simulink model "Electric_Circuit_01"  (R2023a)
settings: Solver=VariableStepAuto  StartTime=0.0  StopTime=10.0  RelTol=1e-3
libraries: fl_lib x8

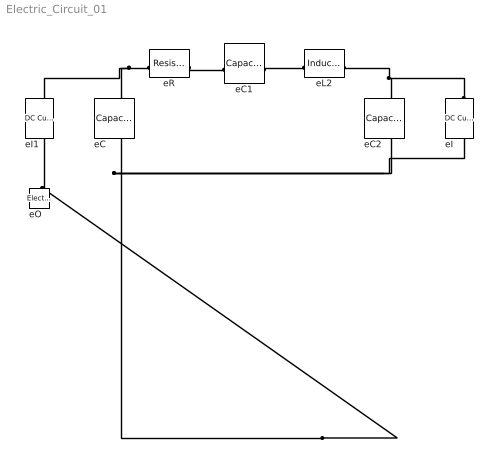
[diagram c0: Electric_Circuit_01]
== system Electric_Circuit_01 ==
  eC : fl_lib/Electrical/Electrical Elements/Capacitor  c=1e-6 F  r=1e-6 Ohm  g=0 1/Ohm  i_specify=off  i_priority=None  i=0 A  i_nominal_specify=off  i_nominal_unit=A  i_nominal_value=1  v_specify=off  v_priority=None  v=0 V  v_nominal_specify=off  v_nominal_unit=V  v_nominal_value=1  vc_specify=off  vc_priority=High  vc=0 V  vc_nominal_specify=off  vc_nominal_unit=V  vc_nominal_value=1
  eC1 : fl_lib/Electrical/Electrical Elements/Capacitor  c=1e-6 F  r=1e-6 Ohm  g=0 1/Ohm  i_specify=off  i_priority=None  i=0 A  i_nominal_specify=off  i_nominal_unit=A  i_nominal_value=1  v_specify=off  v_priority=None  v=0 V  v_nominal_specify=off  v_nominal_unit=V  v_nominal_value=1  vc_specify=off  vc_priority=High  vc=0 V  vc_nominal_specify=off  vc_nominal_unit=V  vc_nominal_value=1
  eC2 : fl_lib/Electrical/Electrical Elements/Capacitor  c=1e-6 F  r=1e-6 Ohm  g=0 1/Ohm  i_specify=off  i_priority=None  i=0 A  i_nominal_specify=off  i_nominal_unit=A  i_nominal_value=1  v_specify=off  v_priority=None  v=0 V  v_nominal_specify=off  v_nominal_unit=V  v_nominal_value=1  vc_specify=off  vc_priority=High  vc=0 V  vc_nominal_specify=off  vc_nominal_unit=V  vc_nominal_value=1
  eI : fl_lib/Electrical/Electrical Sources/DC Current Source  i0=1 A
  eI1 : fl_lib/Electrical/Electrical Sources/DC Current Source  i0=1 A
  eL2 : fl_lib/Electrical/Electrical Elements/Inductor  l=1e-6 H  r=0 Ohm  g=1e-9 1/Ohm  i_specify=off  i_priority=None  i=0 A  i_nominal_specify=off  i_nominal_unit=A  i_nominal_value=1  v_specify=off  v_priority=None  v=0 V  v_nominal_specify=off  v_nominal_unit=V  v_nominal_value=1  i_L_specify=off  i_L_priority=High  i_L=0 A  i_L_nominal_specify=off  i_L_nominal_unit=A  i_L_nominal_value=1
  eO : fl_lib/Electrical/Electrical Elements/Electrical Reference
  eR : fl_lib/Electrical/Electrical Elements/Resistor  R=1 Ohm  i_specify=off  i_priority=None  i=0 A  i_nominal_specify=off  i_nominal_unit=A  i_nominal_value=1  v_specify=off  v_priority=None  v=0 V  v_nominal_specify=off  v_nominal_unit=V  v_nominal_value=1
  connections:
  eO/LConn1 -- eI1/RConn1 -- eC2/RConn1 -- eI/RConn1 -- eC/RConn1
  eR/LConn1 -- eI1/LConn1 -- eC/LConn1
  eI/LConn1 -- eC2/LConn1 -- eL2/RConn1
  eR/RConn1 -- eC1/LConn1
  eC1/RConn1 -- eL2/LConn1
